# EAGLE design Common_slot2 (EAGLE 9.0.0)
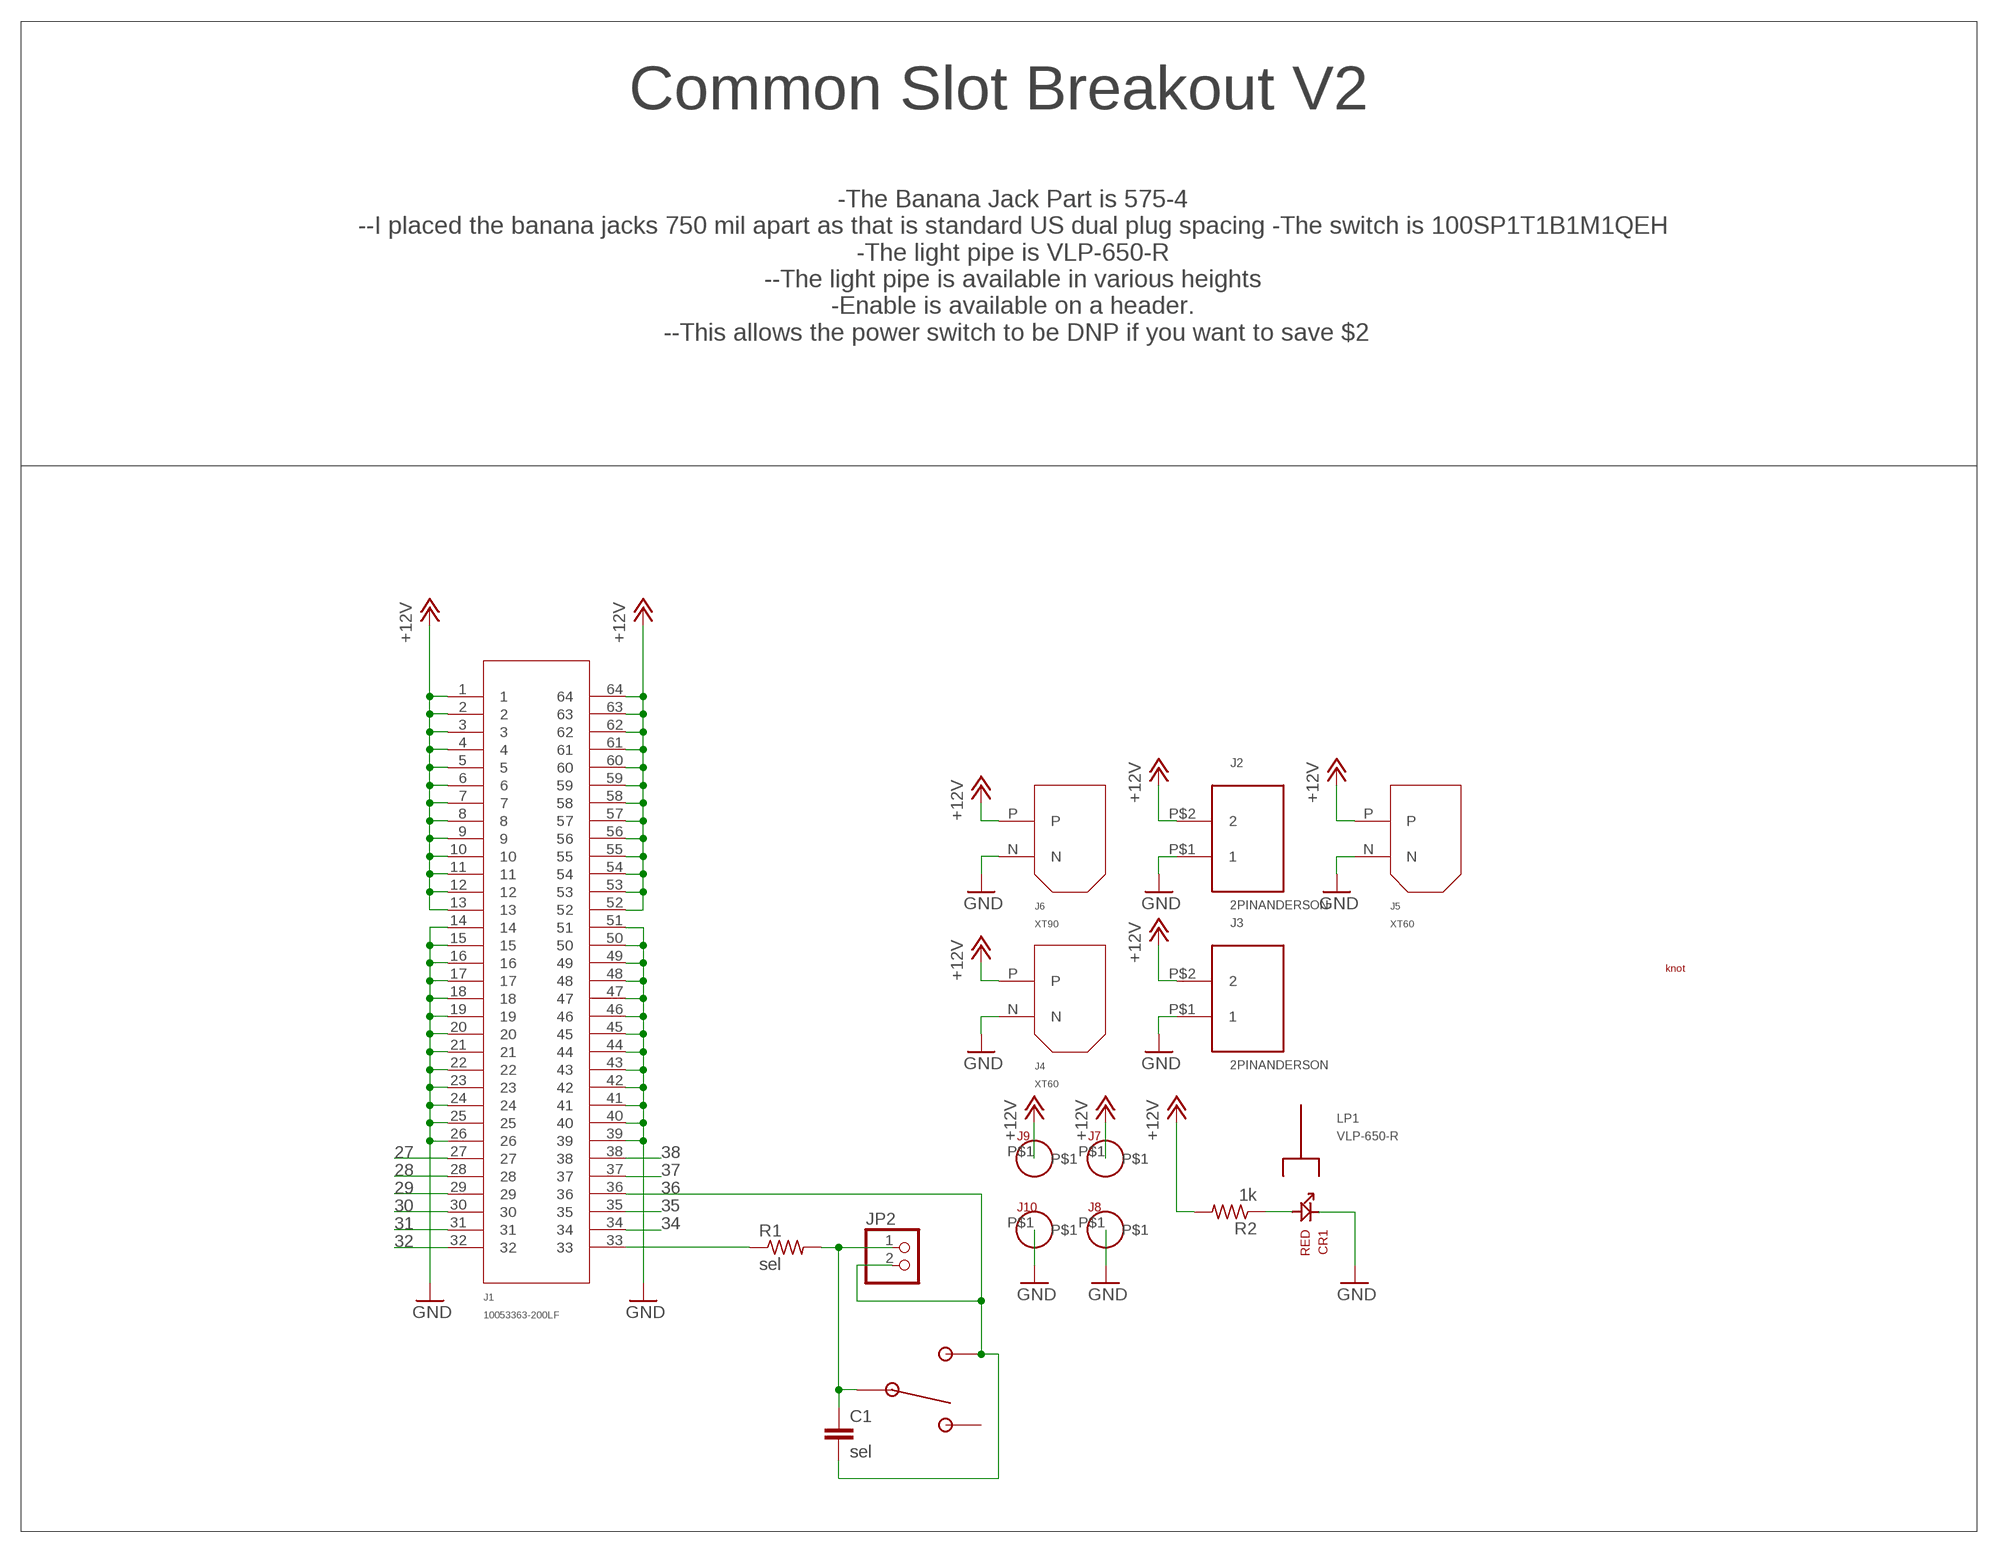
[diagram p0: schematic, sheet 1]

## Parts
C1  sel  0603_CAPACITOR  [0603]
CR1  RED  150060RS75000  [0603_DIODE]
J1  10053363-200LF  [10053363-200LF]
J2  2PINANDERSON  [APP]
J3  2PINANDERSON  [APP]
J4  XT60  [XT60]
J5  XT60  [XT60]
J6  XT90  [XT90]
J7  BANANA  [BANANA]
J8  BANANA  [BANANA]
J9  BANANA  [BANANA]
J10  BANANA  [BANANA]
JP2  PINHD-1X2  [1X02]
LP1  VLP-650-R  [VLP-XXX-R]
R1  sel  0603_RESISTOR  [0603]
R2  1k  0603_RESISTOR  [0603]
SW1  100SP1T1B1M1QEH  [100SP1T1B1M1QEH]
U$1  THIEF_FULL  [THIEF_KNOT]

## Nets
27: J1.27
28: J1.28
29: J1.29
30: J1.30
31: J1.31
32: J1.32
34: J1.34
35: J1.35
36: C1.2 J1.36 JP2.2 SW1.2
37: J1.37
38: J1.38
+12V: J1.1 J1.2 J1.3 J1.4 J1.5 J1.6 J1.7 J1.8 J1.9 J1.10 J1.11 J1.12 J1.13 J1.52 J1.53 J1.54 J1.55 J1.56 J1.57 J1.58 J1.59 J1.60 J1.61 J1.62 J1.63 J1.64 J2.P$2 J3.P$2 J4.P J5.P J6.P J7.P$1 J9.P$1 R2.2
GND: CR1.K J1.14 J1.15 J1.16 J1.17 J1.18 J1.19 J1.20 J1.21 J1.22 J1.23 J1.24 J1.25 J1.26 J1.39 J1.40 J1.41 J1.42 J1.43 J1.44 J1.45 J1.46 J1.47 J1.48 J1.49 J1.50 J1.51 J2.P$1 J3.P$1 J4.N J5.N J6.N J8.P$1 J10.P$1
N$1: J1.33 R1.1
N$2: CR1.A R2.1
N$3: C1.1 JP2.1 R1.2 SW1.C(COM)
Unconnected: SW1.1

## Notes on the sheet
- Common Slot Breakout V2
- -The Banana Jack Part is 575-4 
  --I placed the banana jacks 750 mil apart as that is standard US dual plug spacing -The switch is 100SP1T1B1M1QEH 
  -The light pipe is VLP-650-R 
  --The light pipe is available in various heights 
  -Enable is available on a header. 
  --This allows the power switch to be DNP if you want to save $2

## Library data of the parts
C1 = ruark2:0603_CAPACITOR: 0603 Capacitor -- WARNING: NO DEFINED VALUE OR PART NUMBER
CR1 = ruark2:150060RS75000: Red 625nm LED Indication - Discrete 2V 0603 (1608 Metric); PARTNO: 732-4978-1-ND
J1 = ruark2:10053363-200LF: 64 (Power) Position Female Connector Non Specified - Dual Edge Gold 0.100" (2.54mm) Black; PARTNO: 609-2861-ND
J2 J3 = ruark2:2PINANDERSON
J4 J5 = ruark2:XT60
J6 = ruark2:XT90
J7-J10 = ruark2:BANANA: JACK NON-INSULATED .218" Banana; PARTNO: 36-575-4-ND
JP2 = pinhead:PINHD-1X2: PIN HEADER
LP1 = ruark2:VLP-650-R: Light Pipe Single Clear Rigid Board Mount, Press Fit; PARTNO: 492-2537-ND
R1 = ruark2:0603_RESISTOR: 0603 Resistor -- WARNING: NO DEFINED PART NUMBER OR VALUE
R2 = ruark2:0603_RESISTOR: 0603 Resistor -- WARNING: NO DEFINED PART NUMBER OR VALUE; VALUE: sel
SW1 = ruark2:100SP1T1B1M1QEH: Toggle Switch SPDT Panel Mount; PARTNO: EG2350-ND
U$1 = ruark2:THIEF_FULL; PARTNO: NA

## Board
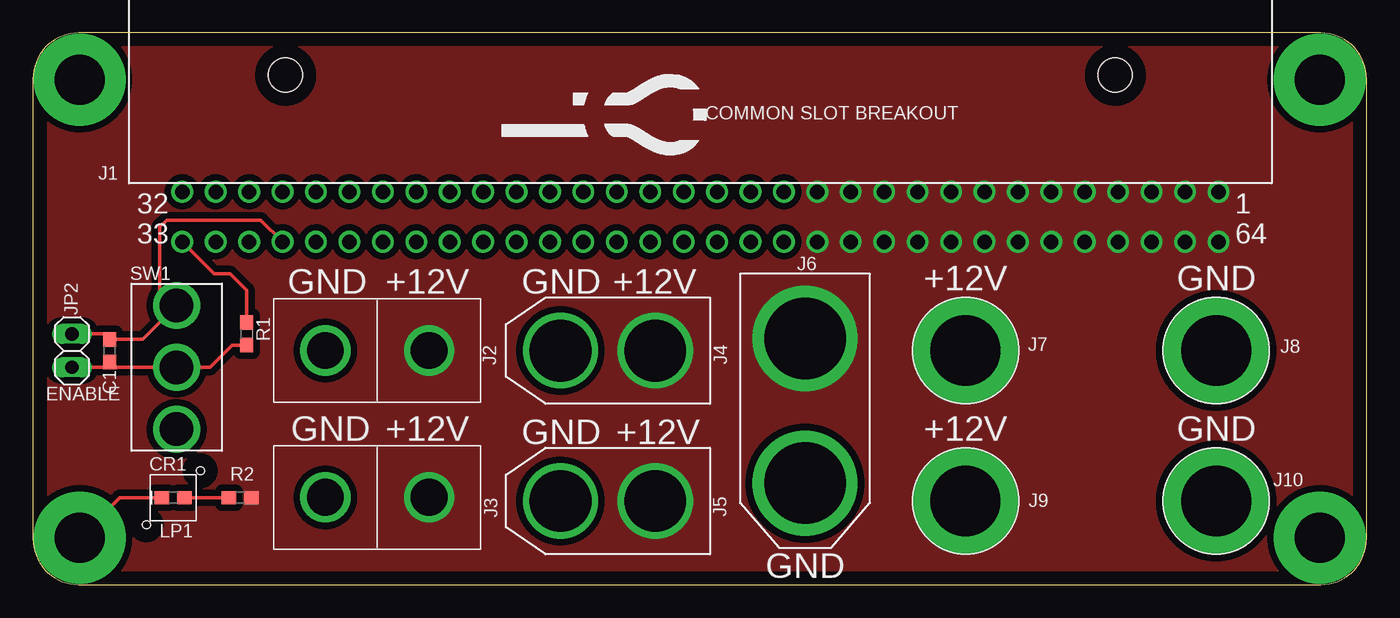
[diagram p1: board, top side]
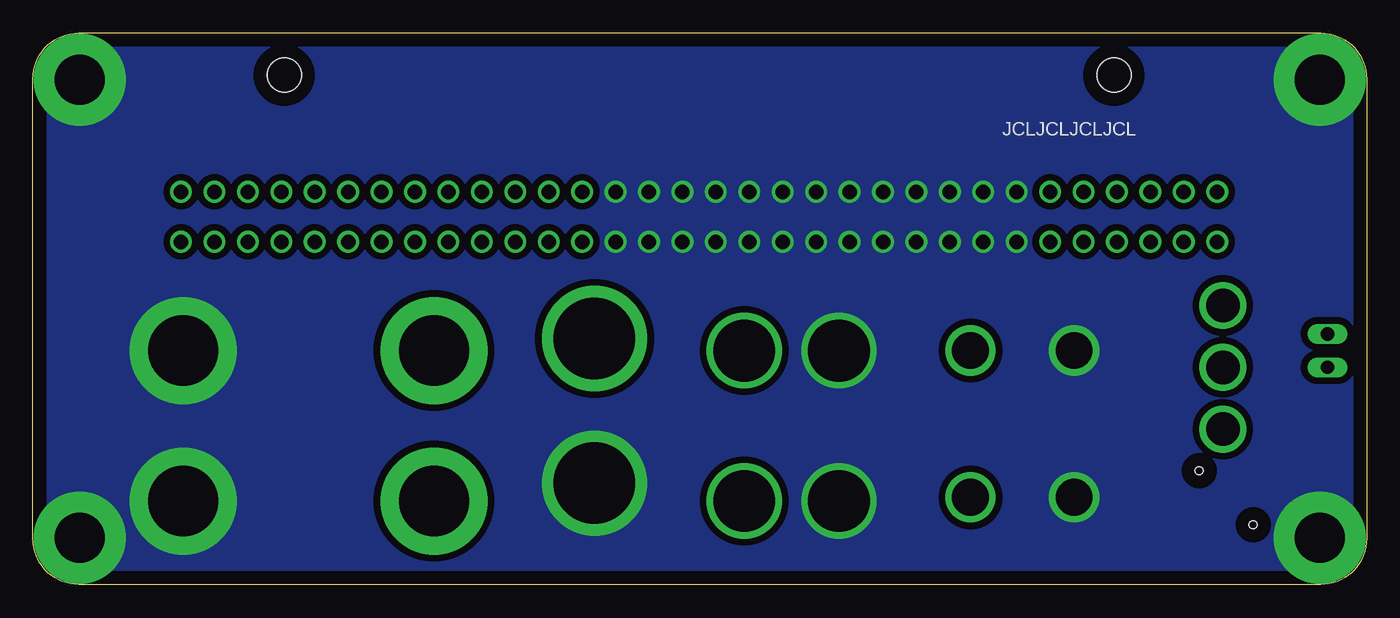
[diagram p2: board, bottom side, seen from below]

Size 101.35 x 41.91 mm. Coordinates in mm from the lower left corner, seen from the top.
Outline: 0,38.42 0,3.49 arc90 3.49,0 97.85,0 arc90 101.35,3.49 101.35,38.42 arc90 97.85,41.91 3.49,41.91 arc90 0,38.42
Copper layers (1*16): Top 0.035mm / dielectric 1.5mm / Bottom 0.035mm
Design rules "default": minimum track width 6mil, minimum drill 0.35mm, track to track 6mil, track to pad 6mil, pad to pad 6mil, via to via 6mil, smd to smd 6mil, copper to edge 40mil, drill to drill 6mil, minimum pad ring 10mil, minimum via ring 8mil, stop-mask expansion 4mil, vias tented up to drill 0mil, thermal gap 10mil

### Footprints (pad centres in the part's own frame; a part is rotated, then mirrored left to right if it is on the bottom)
0603 = smd 1.1 x 1: 1 -0.85,0; 2 0.85,0
0603_DIODE = smd 1.1 x 1: A -0.85,0; K 0.85,0
10053363-200LF = drill 1.1: 1 39.37,1.9; 2 36.83,1.9; 3 34.29,1.9; 4 31.75,1.9; 5 29.21,1.9; 6 26.67,1.9; 7 24.13,1.9; 8 21.59,1.9; 9 19.05,1.9; 10 16.51,1.9; 11 13.97,1.9; 12 11.43,1.9; 13 8.89,1.9; 14 6.35,1.9; 15 3.81,1.9; 16 1.27,1.9; 17 -1.27,1.9; 18 -3.81,1.9; 19 -6.35,1.9; 20 -8.89,1.9; 21 -11.43,1.9; 22 -13.97,1.9; 23 -16.51,1.9; 24 -19.05,1.9; 25 -21.59,1.9; 26 -24.13,1.9; 27 -26.67,1.9; 28 -29.21,1.9; 29 -31.75,1.9; 30 -34.29,1.9; 31 -36.83,1.9; 32 -39.37,1.9; 33 -39.37,-1.9; 34 -36.83,-1.9; 35 -34.29,-1.9; 36 -31.75,-1.9; 37 -29.21,-1.9; 38 -26.67,-1.9; 39 -24.13,-1.9; 40 -21.59,-1.9; 41 -19.05,-1.9; 42 -16.51,-1.9; 43 -13.97,-1.9; 44 -11.43,-1.9; 45 -8.89,-1.9; 46 -6.35,-1.9; 47 -3.81,-1.9; 48 -1.27,-1.9; 49 1.27,-1.9; 50 3.81,-1.9; 51 6.35,-1.9; 52 8.89,-1.9; 53 11.43,-1.9; 54 13.97,-1.9; 55 16.51,-1.9; 56 19.05,-1.9; 57 21.59,-1.9; 58 24.13,-1.9; 59 26.67,-1.9; 60 29.21,-1.9; 61 31.75,-1.9; 62 34.29,-1.9; 63 36.83,-1.9; 64 39.37,-1.9 | hole 2.6: -31.52,10.76; 31.52,10.76
APP = drill 2.794: P$1 3.937,0; P$2 -3.937,0
XT60 = drill 4.7: N 0,3.6; P 0,-3.6
XT90 = drill 6.2 pad 8: N 0,5.5; P 0,-5.5
BANANA = drill 5.334 pad 8.128: P$1 0,0
1X02 = drill 1.016 long: 1 -1.27,0; 2 1.27,0
VLP-XXX-R = hole 0.61: 2.05,2.05; -2.05,-2.05
100SP1T1B1M1QEH = drill 2.54: 1 0,4.699; 2 0,-4.699; C 0,0

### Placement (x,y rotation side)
C1  5.84,17.78 90 top
CR1  10.67,6.6 180 top
J1  50.72,27.94 0 top
J2  26.16,17.78 180 top
J3  26.16,6.63 180 top
J4  43.69,17.78 90 top
J5  43.69,6.35 90 top
J6  58.67,13.21 180 top
J7  70.87,17.78 0 top
J8  89.92,17.78 0 top
J9  70.87,6.35 0 top
J10  89.92,6.35 0 top
JP2  2.97,17.78 90 top
LP1  10.67,6.6 0 top
R1  16.26,19.05 270 top
R2  15.75,6.6 0 top
SW1  10.92,16.51 180 top
U$1  34.8,30.99 0 top

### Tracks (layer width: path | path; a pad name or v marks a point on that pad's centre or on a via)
36
  Top 0.254: JP2.2 5.42,19.05 C1.2 8.34,18.63 10.86,21.14 | 10.86,21.14 SW1.2 | J1.36 17.32,27.69 10.16,27.69 9.65,27.18 9.65,22.35 10.86,21.14
+12V
  pour Top (isolate 0.508, no thermals): 0.51,0 0.51,41.91 100.33,41.91 100.33,0
GND  (via drill 3.81 pad 6.99)
  Top 0.254: CR1.K 6.6,6.6 v3.56,3.56
  other vias: 3.56,38.35 97.79,38.35 97.79,3.56
  pour Bottom (isolate 0.508, no thermals): 0.76,0 0.76,41.91 100.33,41.91 100.33,0
N$1
  Top 0.254: R1.1 16.26,22.35 14.99,23.62 13.77,23.62 J1.33
N$2
  Top 0.254: R2.1 CR1.A
N$3
  Top 0.254: 16.31,18.15 R1.2 15.15,18.2 13.46,16.51 SW1.C 5.84,16.51 | 5.84,16.51 JP2.1 | C1.1 5.84,16.51

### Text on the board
tPlace: GND | +12V | GND | +12V | +12V | GND | GND | +12V | GND | +12V | +12V | GND | GND
tNames: COMMON SLOT BREAKOUT | ENABLE
bNames: JCLJCLJCLJCL
tStop: MMXX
